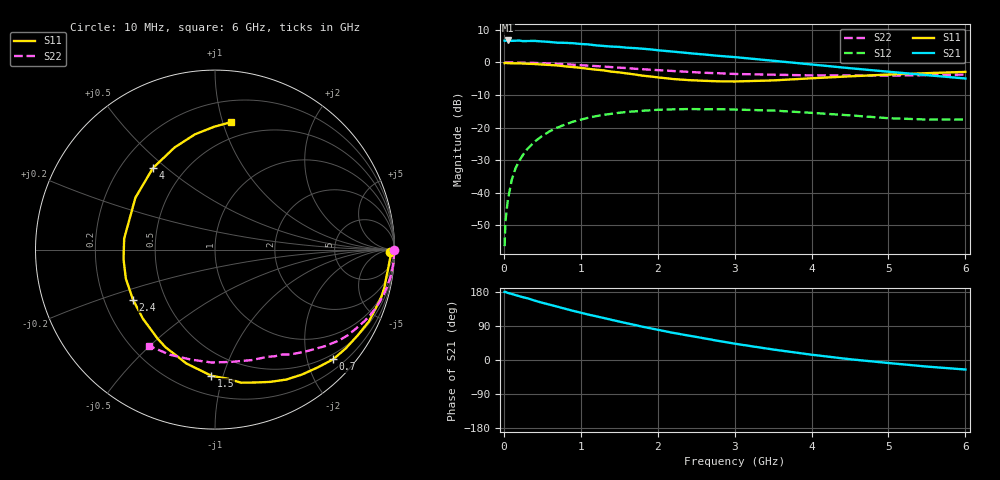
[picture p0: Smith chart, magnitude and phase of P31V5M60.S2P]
! SIEMENS Small Signal Semiconductors
! BFP181
! Si NPN RF Bipolar Junction Transistor in SOT143
! VCE = 1.5 V  IC = 0.6 mA
! Common Emitter S-Parameters:  March  1996
# GHz  S  MA  R  50
!  f  S11  S21  S12  S22
! GHz  MAG  ANG  MAG  ANG  MAG  ANG  MAG  ANG
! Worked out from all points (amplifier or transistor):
!   36 points, 10 MHz to 6 GHz, reference 50 ohm
!   highest |S21| = 6.8 dB at 50 MHz (marker M1)
!   |S21| within 3 dB of that: start of sweep to 1.998 GHz
!   unconditionally stable (mu >= 1): 3.566 GHz to end of sweep
!   at 250 MHz: K = 0.08, MSG = 17.5 dB, |S12| = -28.4 dB
!   at 1.4 GHz: K = 0.46, MSG = 10.3 dB, |S12| = -15.8 dB
!   at 6 GHz: K = 1.45, MAG = 2.3 dB, |S12| = -17.6 dB
!   S11 on the Smith chart (normalised r, x): 10 MHz: 60, -33; 700 MHz: 0.39, -2.49; 1.5 GHz: 0.33, -0.92; 2.4 GHz: 0.32, -0.25; 4 GHz: 0.33, +0.45; 6 GHz: 0.37, +1.07
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0.01  0.9748 -0.8  2.159 179.7  0.0015 87.4  0.9998 -0.2
0.02  0.9816 -1.3  2.156 179.6  0.0035 83.6  0.9999 -0.6
0.05  0.9769 -2.8  2.178 177.2  0.0074 90.0  0.9976 -1.5
0.1  0.9705 -6.3  2.148 174.4  0.0152 85.4  0.9971 -3.0
0.15  0.9669 -9.5  2.156 171.4  0.0234 82.7  0.9962 -4.5
0.2  0.9672 -12.5  2.174 168.4  0.0307 81.2  0.9942 -6.0
0.25  0.9637 -15.6  2.128 165.6  0.0382 79.4  0.9904 -7.6
0.4  0.9465 -25.0  2.143 156.8  0.0606 72.7  0.9818 -11.9
0.5  0.9276 -31.0  2.102 151.0  0.0745 68.1  0.9732 -14.9
0.7  0.8985 -42.9  2.009 140.5  0.1003 60.2  0.9502 -20.5
0.9  0.8481 -55.2  1.977 129.7  0.1228 52.2  0.923 -25.6
1.1  0.7984 -67.4  1.893 119.8  0.1414 44.9  0.8931 -30.5
1.5  0.7034 -91.6  1.734 101.4  0.1685 31.9  0.8316 -39.1
1.8  0.6272 -110.4  1.628 87.9  0.1809 23.8  0.7875 -44.5
2.2  0.5565 -136.1  1.467 71.6  0.1902 13.7  0.7385 -51.3
2.4  0.5353 -148.6  1.392 64.5  0.1923 9.2  0.7172 -54.6
3  0.5098 173.1  1.209 43.1  0.1886 -2.1  0.6655 -63.8
3.5  0.5294 146.9  1.062 27.7  0.1825 -9.0  0.6484 -71.7
4  0.571 127.3  0.931 14.0  0.168 -14.3  0.6325 -81.2
4.5  0.6119 111.6  0.816 2.0  0.1538 -17.9  0.6295 -91.6
5.5  0.6845 90.4  0.638 -17.4  0.1326 -14.4  0.6377 -113.4
6  0.716 82.8  0.567 -25.1  0.1325 -10.9  0.6503 -124.7
